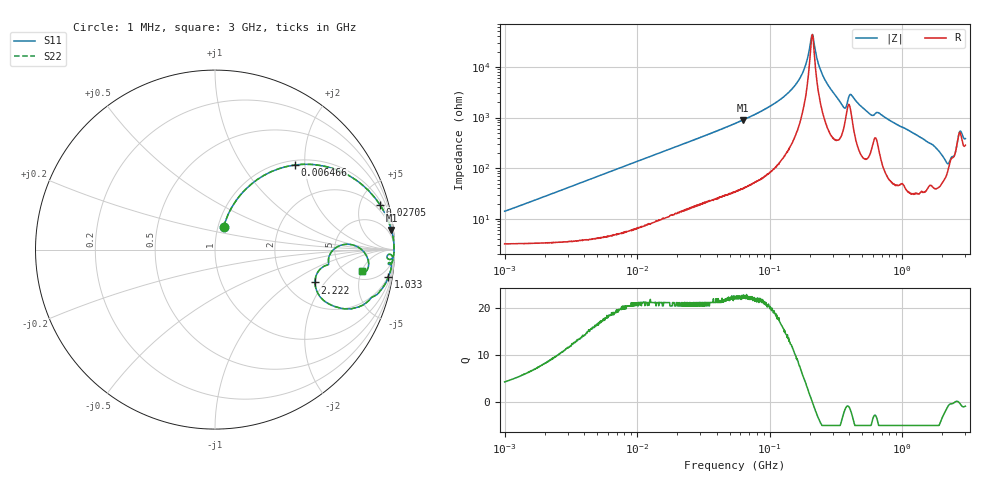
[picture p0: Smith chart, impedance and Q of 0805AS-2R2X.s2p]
!s-Parameter Generated by FASTRON Sdn. Bhd.
!FASTRON P/N : 0805AS-2R2X
!Keysight Technologies: E4991B_MY54100416_A.01.15
!Date: Mon Jun 15 12:57:41 2026
!Version  :Rev01  Mon Jun 15 12:57:41 2026
!Data & Calibration Information:
!Freq  S11  S21  S12  S22
!PortZ  Port1:50+j0  Port2:50+j0
!When reading reference impedance value at option line is always used.
! Remarks : This data is being provided solely for informational purposes.
# Hz S dB R 50
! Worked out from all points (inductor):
!   1601 points, 1 MHz to 3 GHz, reference 50 ohm
!   read as one part in series: L = 2.19 uH near 1.041 MHz
!   highest Q = 22.5 at 63.01 MHz (marker M1), where L = 2.25 uH
!   self-resonance near 209.4 MHz
!   S11 on the Smith chart (normalised r, x): 1 MHz: 1.06, +0.28; 6.466 MHz: 1.10, +1.77; 27.05 MHz: 1.35, +7.30; 1.033 GHz: 2, -12; 2.222 GHz: 2.86, -1.60; 3 GHz: 6.70, -5.13
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1000000  -17.30 69.2  -0.35 -7.6  -0.35 -7.6  -17.30 69.2
3804036  -6.92 59.1  -1.30 -26.7  -1.30 -26.7  -6.92 59.1
6465526  -3.79 46.7  -2.74 -40.2  -2.74 -40.2  -3.79 46.7
1.447069e7  -1.16 26.4  -7.04 -60.9  -7.04 -60.9  -1.16 26.4
2.704826e7  -0.42 15.1  -11.70 -72.1  -11.70 -72.1  -0.42 15.1
5.504702e7  -0.12 7.4  -17.80 -80.1  -17.80 -80.1  -0.12 7.4
6.301011e7  -0.10 6.3  -19.10 -81.1  -19.10 -81.1  -0.10 6.3
1.103592e8  -0.04 2.9  -25.80 -84.0  -25.80 -84.0  -0.04 2.9
1.505037e8  -0.02 1.5  -31.90 -83.4  -31.90 -83.4  -0.02 1.5
1.820241e8  -0.02 0.6  -39.10 -77.8  -39.10 -77.8  -0.02 0.6
2.083556e8  -0.02 0.0  -52.50 -14.4  -52.50 -14.4  -0.02 0.0
2.519921e8  -0.02 -0.8  -36.60 78.8  -36.60 78.8  -0.02 -0.8
3.55908e8  -0.17 -3.2  -24.80 69.1  -24.80 69.1  -0.17 -3.2
4.114912e8  -0.14 -1.8  -29.20 62.4  -29.20 62.4  -0.14 -1.8
5.696638e8  -0.14 -4.7  -21.60 76.2  -21.60 76.2  -0.14 -4.7
7.925923e8  -0.12 -6.3  -19.20 79.9  -19.20 79.9  -0.12 -6.3
1.033307e9  -0.21 -9.0  -16.10 76.9  -16.10 76.9  -0.21 -9.0
1.950859e9  -1.74 -23.8  -7.64 52.8  -7.64 52.8  -1.74 -23.8
2.221924e9  -4.63 -18.2  -6.39 22.4  -6.39 22.4  -4.63 -18.2
2.543347e9  -3.16 1.8  -10.30 -4.1  -10.30 -4.1  -3.16 1.8
2.727913e9  -1.43 -2.8  -16.00 15.2  -16.00 15.2  -1.43 -2.8
3e9  -1.63 -8.3  -13.30 33.7  -13.30 33.7  -1.63 -8.3
